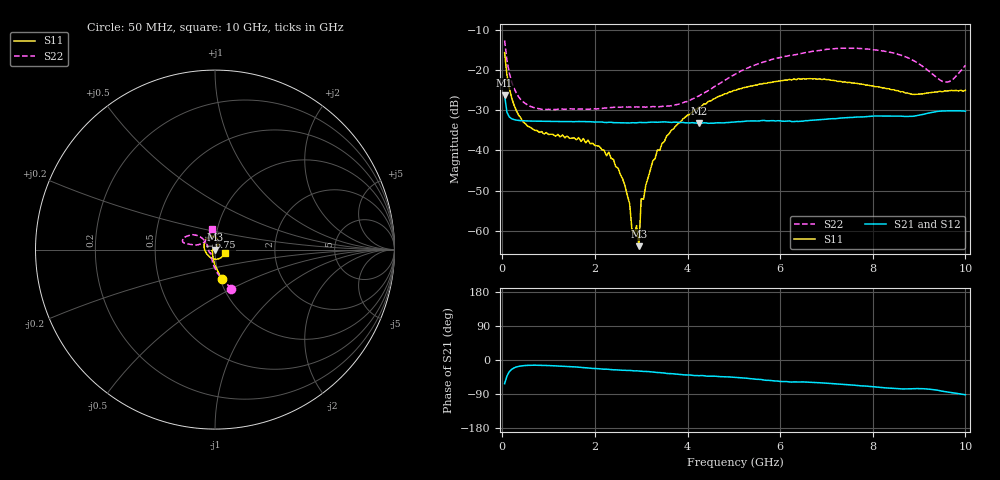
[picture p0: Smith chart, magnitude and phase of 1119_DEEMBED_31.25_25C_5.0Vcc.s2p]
!Hittite Microwave Corp.
!Digital Attenuator/PhaseShifter Rev 1.4.0
!Filename: C:\DATA\DATA\1119_DEEMBED_31.25_25C_5.0Vcc.s2p
!VNA ID: Agilent Technologies,N5224A,MY51441122,A.10.45.03
!Device type:
!2 Port Calibration.
!Temp(C): 25
!Lot Number:
!Serial Number:
!Operator:
!Misc:
!Attenuator:  31.250
# GHZ S DB R 50.0
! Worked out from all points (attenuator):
!   200 points, 50 MHz to 10 GHz, reference 50 ohm
!   highest |S21| = -26.27 dB at 50 MHz (marker M1); lowest = -33.2 dB at 4.25 GHz (marker M2)
!   lowest |S11| = -63.9 dB at 2.95 GHz (marker M3), VSWR 1.00, Z = 50 - j0.0485 ohm
!   |S11| at or under -10 dB: start of sweep to end of sweep
!   |S22| runs from -29.8 to -12.6 dB; largest |S21 - S12| = 8.9e-05
!   S11 on the Smith chart (normalised r, x): 50 MHz: 1.02, -0.34; 6.75 GHz: 0.92, +0.13; 10 GHz: 1.11, -0.04
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0.05  -15.60 -77.3  -26.27 -62.5  -26.27 -62.6  -12.56 -67.6
0.1  -21.15 -90.2  -30.45 -42.4  -30.44 -42.5  -17.51 -84.0
0.2  -26.78 -104.1  -32.07 -24.9  -32.06 -24.9  -22.78 -100.6
0.45  -32.89 -126.7  -32.59 -15.0  -32.58 -14.9  -27.86 -121.4
1.75  -37.03 -162.5  -32.80 -20.1  -32.82 -20.2  -29.67 -140.9
2.3  -40.42 -167.2  -32.96 -24.7  -32.96 -24.7  -29.30 -149.4
2.5  -44.36 -163.3  -33.09 -26.3  -33.09 -26.3  -29.20 -151.6
2.75  -53.29 -160.1  -33.14 -27.6  -33.14 -27.7  -29.16 -155.6
2.8  -59.78 -108.4  -33.07 -27.9  -33.08 -28.0  -29.16 -156.7
2.9  -58.74 -2.6  -33.11 -28.5  -33.12 -28.7  -29.12 -159.2
2.95  -63.86 -49.1  -33.01 -28.9  -33.02 -29.0  -29.15 -160.3
3  -52.02 21.6  -33.01 -29.6  -33.02 -29.7  -29.12 -161.8
3.05  -52.13 26.5  -33.05 -30.1  -33.05 -30.2  -29.17 -163.1
3.25  -42.58 40.0  -32.92 -31.9  -32.94 -32.0  -29.03 -169.0
3.4  -39.97 49.2  -32.93 -33.1  -32.95 -33.2  -29.06 -173.9
4.25  -29.18 57.2  -33.23 -41.4  -33.23 -41.5  -26.38 152.0
5.05  -24.95 73.6  -32.87 -45.9  -32.89 -46.0  -20.83 138.5
6.7  -22.15 116.0  -32.45 -59.2  -32.45 -59.2  -15.27 153.8
6.75  -22.10 116.7  -32.42 -59.6  -32.43 -59.6  -15.19 154.4
8.35  -24.61 178.7  -31.42 -74.0  -31.43 -74.0  -15.45 168.1
9.55  -25.13 -70.7  -30.13 -83.3  -30.14 -83.3  -22.91 138.0
10  -25.00 -19.4  -30.20 -91.7  -30.21 -91.7  -18.77 98.2
